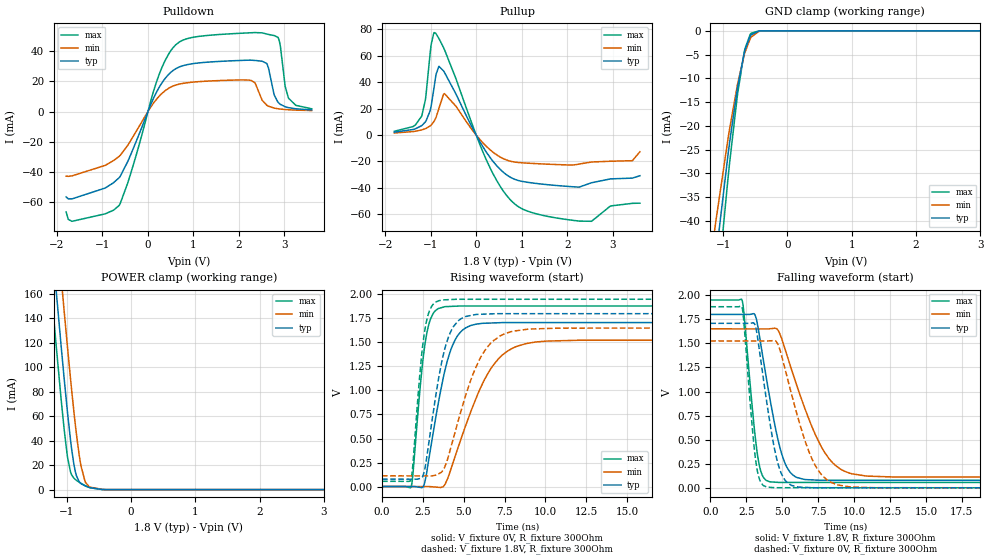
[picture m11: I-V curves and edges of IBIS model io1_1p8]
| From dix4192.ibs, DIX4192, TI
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|   io1_1p8 Model
[Model]   io1_1p8
Model_type   I/O
Polarity   Non-Inverting
Enable   Active-Low
Vinl = 0.54
Vinh = 1.26
Vmeas = 0.9
Vref = 0
Cref = 2pF
Rref = 100000
|   typ   min   max
C_comp   31.1632pF   25.3303pF   36.9522pF
|C_comp_pullup   31.8884pF   25.9187pF   37.6383pF
|C_comp_pulldown   31.5964pF   25.8002pF   37.4615pF
[Model spec]
|subparameter
Vinl   0.54   0.495   0.585
Vinh   1.26   1.155   1.365
| Where nom  PVT is Nominal Process, 1.8V, 27C
|   Fast PVT is Strong Process,  1.95V, -40C
|   Slow PVT is Weak Process,   1.65V, 105C
[Voltage Range]   1.8   1.65   1.95
[Temperature Range]   27   105   -40
[Pullup Reference]   1.8   1.65   1.95
[Pulldown Reference]   0   0   0
[Power Clamp Reference]   1.8   1.65   1.95
[GND Clamp Reference]   0   0   0
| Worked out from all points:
|   slope of the pulldown table from 0 to 0.27 V, typ, clamps not added: 15.7 ohm
|   slope of the pullup table from 0 to 0.27 V, typ, clamps not added: 17.7 ohm
|   GND clamp passes 1 mA (typ) near -0.57 V on its own axis
|   POWER clamp passes 1 mA (typ) near -0.56 V on its own axis
|   falling waveform, V_fixture 1.8V, R_fixture 300Ohm: 20-80 % time 1.29ns typ, 2.34ns min, 720ps max; typ from 1.8 V to 0.077 V
|   rising waveform, V_fixture 0V, R_fixture 300Ohm: 20-80 % time 1.18ns typ, 2.18ns min, 638ps max; typ from 0 V to 1.71 V
|   rising waveform, V_fixture 1.8V, R_fixture 300Ohm: 20-80 % time 1.04ns typ, 1.8ns min, 589ps max; typ from 0.077 V to 1.8 V
|   falling waveform, V_fixture 0V, R_fixture 300Ohm: 20-80 % time 1.08ns typ, 1.84ns min, 635ps max; typ from 1.71 V to 0 V
[Pulldown]
|   Voltage   I(typ)   I(min)   I(max)
-1.8V     -56.63mA   -42.81mA   -66.55mA
-1.67V    -57.92mA   -42.67mA   -72.79mA
-633.6mV  -43.88mA   -29.73mA   -62.29mA
273.6mV   17.4mA     10.99mA    26.7mA
765mV     30.33mA    18.63mA    47.27mA
2.266V    34.03mA    20.63mA    52.22mA
2.509V    33.35mA    7.565mA    52.15mA
2.617V    31.56mA    4.064mA    51.33mA
2.855V    6.344mA    1.84mA     49.25mA
3.017V    3.179mA    1.318mA    16.68mA
3.087V    2.59mA     1.171mA    9.115mA
3.6V      1.075mA    640.9uA    1.804mA
[GND Clamp]
|   Voltage   I(typ)   I(min)   I(max)
-1.8V     -142.7mA   -115.7mA   -175.3mA
-1.168V   -54.5mA    -45.47mA   -65.99mA
-1.114V   -47.82mA   -40.13mA   -57.84mA
-1.109V   -47.17mA   -39.6mA    -57.04mA
-925.2mV  -26.15mA   -22.77mA   -31.1mA
-779.4mV  -12.17mA   -11.45mA   -13.67mA
-666mV    -4.303mA   -4.77mA    -4.076mA
-579.6mV  -1.122mA   -1.659mA   -756.7uA
-563.4mV  -812.7uA   -1.293mA   -503.6uA
-444.6mV  -43.31uA   -131.8uA   -12uA
-342mV    -1.686uA   -11.57uA   -47.06nA
3.6V      0A         0A         0A
[Pullup]
|   Voltage   I(typ)   I(min)   I(max)
-1.8V     2.198mA    1.55mA     2.867mA
-1.201V   7.084mA    3.863mA    14.25mA
-1.114V   10.13mA    4.875mA    27.64mA
-1.017V   18.04mA    6.818mA    60.52mA
-925.2mV  36.38mA    10.47mA    77.67mA
-822.6mV  51.95mA    19.8mA     73.34mA
-698.4mV  47.53mA    31.43mA    64.82mA
235.8mV   -13.6mA    -8.983mA   -19.78mA
840.6mV   -33.45mA   -20.44mA   -52.05mA
2.536V    -36.14mA   -20.43mA   -65.37mA
2.952V    -33.23mA   -19.83mA   -53.75mA
3.6V      -30.86mA   -12.67mA   -51.62mA
[POWER Clamp]
|   Voltage   I(typ)   I(min)   I(max)
-1.8V     564.8mA    620.9mA    520.8mA
-1.233V   204.8mA    261.9mA    159.6mA
-1.168V   165.5mA    222.3mA    120.5mA
-1.087V   117.7mA    173.8mA    74.13mA
-1.039V   90.27mA    145.4mA    48.83mA
-984.6mV  61.6mA     114.7mA    25.82mA
-941.4mV  40.98mA    91.12mA    14.65mA
-887.4mV  20.49mA    63.43mA    9.326mA
-806.4mV  6.463mA    28.45mA    6.043mA
-714.6mV  3.048mA    6.727mA    3.292mA
-412.2mV  29.86uA    75.2uA     8.811uA
3.6V      0A         0A         0A
[Ramp]
R_load = 300
|   typ   min   max
dV/dt_r   1.02457/1.17895e-09   0.914694/2.1782e-09   1.12794/6.37688e-10
dV/dt_f   1.03368/1.28526e-09   0.923167/2.34361e-09   1.13713/7.1709e-10
[Falling Waveform]
V_fixture = 1.8V
V_fixture_min = 1.65V
V_fixture_max = 1.95V
R_fixture = 300Ohm
C_fixture = 0F
|   Time   V(typ)   V(min)   V(max)
0s        1.8V       1.65V      1.95V
2.211ns   1.8V       1.65V      1.948V
3.05ns    1.806V     1.65V      635.2mV
3.304ns   1.678V     1.65V      322.3mV
4.133ns   937.5mV    1.651V     62.91mV
4.77ns    462.1mV    1.622V     56.31mV
5.598ns   154.5mV    1.252V     56.07mV
7.757ns   78.46mV    417.2mV    56.07mV
9.864ns   78.46mV    145.3mV    56.06mV
50ns      77.2mV     111.4mV    54.79mV
[Rising Waveform]
V_fixture = 0V
V_fixture_min = 0V
V_fixture_max = 0V
R_fixture = 300Ohm
C_fixture = 0F
|   Time   V(typ)   V(min)   V(max)
0s        -427.5nV   -61.84nV   -730.2nV
1.774ns   107uV      58.07uV    -5.9mV
2.507ns   -4.739mV   82.08uV    1.325V
2.755ns   171.3mV    90.21uV    1.61V
3.178ns   609.9mV    -3.851mV   1.813V
3.843ns   1.205V     20.61mV    1.872V
4.787ns   1.605V     473.7mV    1.879V
6.513ns   1.701V     1.187V     1.879V
8.885ns   1.706V     1.49V      1.879V
50ns      1.708V     1.524V     1.88V
[Rising Waveform]
V_fixture = 1.8V
V_fixture_min = 1.65V
V_fixture_max = 1.95V
R_fixture = 300Ohm
C_fixture = 0F
|   Time   V(typ)   V(min)   V(max)
0s        77.2mV     111.4mV    54.79mV
1.768ns   76.7mV     110.9mV    72.46mV
2.31ns    83.06mV    110.8mV    1.166V
2.607ns   173.3mV    110.7mV    1.617V
3.018ns   639.6mV    110.6mV    1.87V
3.673ns   1.313V     156.4mV    1.941V
4.625ns   1.718V     662.4mV    1.949V
5.957ns   1.792V     1.319V     1.949V
8.03ns    1.799V     1.617V     1.949V
50ns      1.8V       1.65V      1.95V
[Falling Waveform]
|Gnd
V_fixture = 0V
V_fixture_min = 0V
V_fixture_max = 0V
R_fixture = 300Ohm
C_fixture = 0F
|   Time   V(typ)   V(min)   V(max)
0s        1.708V     1.524V     1.88V
2.201ns   1.707V     1.524V     1.877V
3.178ns   1.654V     1.524V     262.8mV
3.459ns   1.381V     1.524V     75.09mV
3.951ns   864.8mV    1.524V     7.318mV
4.625ns   298.6mV    1.51V      1.313mV
5.249ns   70.76mV    1.204V     1.312mV
7.085ns   1.864mV    296.6mV    1.31mV
8.885ns   1.14mV     29.68mV    1.307mV
50ns      -135.5nV   -60.92nV   -730.5nV
